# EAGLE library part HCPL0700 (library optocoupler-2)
HEWLETT PACKARD OPTO COUPLER
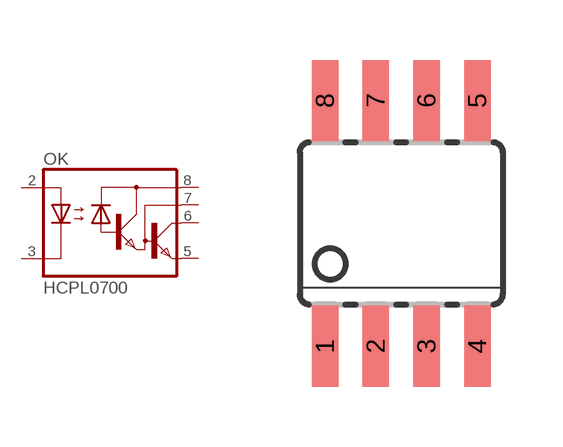
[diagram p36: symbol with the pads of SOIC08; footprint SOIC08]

Designator prefix OK

## HCPL0700  [SOIC08]
2  A  pas
3  C  pas
5  GND  pas
6  VO  pas
7  VB  pas
8  VCC  pas

## Footprint SOIC08 (pad centres in mm)
Small Outline Package
smd 0.66 x 2.032: 1 -1.905,-3.073; 2 -0.635,-3.073; 3 0.635,-3.073; 4 1.905,-3.073; 5 1.905,3.073; 6 0.635,3.073; 7 -0.635,3.073; 8 -1.905,3.073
